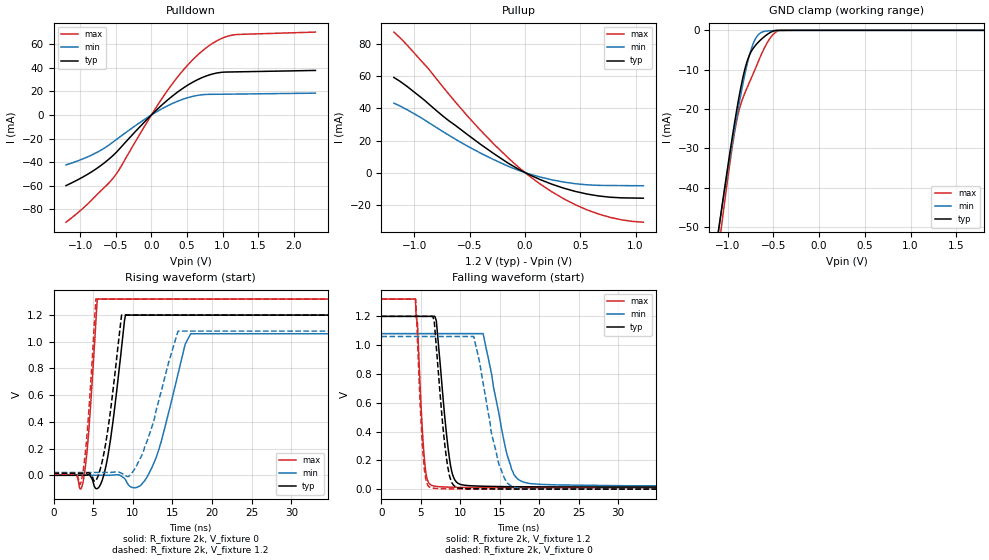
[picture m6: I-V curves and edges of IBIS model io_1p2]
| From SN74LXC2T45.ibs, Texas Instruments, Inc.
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[Model]   io_1p2
Model_type  I/O
Vinl=0.3
Vinh=0.9
Enable   Active-Low
Vref =   0
Rref =   2000
Cref =   15p
Vmeas =   0.6
| variable   typ   min   max
C_comp   6.34pF   5.61pF   7.15pF
| C_pullup   10.74pF   6.64pF   16.31pF
| C_pulldown   10.09pF   6.99pF   16.46pF
| C_tri-state   6.34pF   5.61pF   7.15pF
[Temperature Range]   25   125   -40
| Ambient temperature   25   85   -40
[Voltage range]   1.2   1.08   1.32
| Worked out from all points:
|   slope of the pulldown table from 0 to 0.18 V, typ, clamps not added: 17.6 ohm
|   slope of the pullup table from 0 to 0.18 V, typ, clamps not added: 32.4 ohm
|   GND clamp passes 1 mA (typ) near -0.56 V on its own axis
|   rising waveform, R_fixture 2k, V_fixture 0: 20-80 % time 1.47ns typ, 2.68ns min, 895ps max; typ from 0 V to 1.2 V
|   falling waveform, R_fixture 2k, V_fixture 1.2: 20-80 % time 1.23ns typ, 2.26ns min, 715ps max; typ from 1.2 V to 0.015 V
|   rising waveform, R_fixture 2k, V_fixture 1.2: 20-80 % time 1.51ns typ, 2.99ns min, 895ps max; typ from 0.015 V to 1.2 V
|   falling waveform, R_fixture 2k, V_fixture 0: 20-80 % time 1.19ns typ, 2.18ns min, 690ps max; typ from 1.2 V to 0 V
[GND Clamp]
| LXC8T245_IO_12
|   Voltage   I(typ)   I(min)   I(max)
-5.5V     -897.1mA   -831.9mA   -1.015A
-1.11V    -52.66mA   -52.33mA   -57.72mA
-1.08V    -47.7mA    -47.75mA   -52.14mA
-1.05V    -42.82mA   -43.24mA   -46.67mA
-915mV    -22.23mA   -23.93mA   -24.75mA
-835mV    -12.18mA   -13.81mA   -17.31mA
-785mV    -7.737mA   -8.436mA   -14.47mA
-735mV    -5.102mA   -4.277mA   -11.79mA
-645mV    -2.561mA   -727uA     -6.848mA
-530mV    -501.4uA   -105.7uA   -1.806mA
-430mV    -5.242uA   -35.39uA   -19.91uA
1.8V      23.18pA    30.38nA    510.2pA
[Pulldown]
| LXC8T245_IO_12
|   Voltage   I(typ)   I(min)   I(max)
-1.2V     -60.02mA   -42.43mA   -91.1mA
-835mV    -48.11mA   -33.91mA   -71.97mA
-655mV    -40.41mA   -27.94mA   -61.23mA
-525mV    -33.63mA   -22.34mA   -52.68mA
-430mV    -27.57mA   -18.06mA   -44.1mA
-110mV    -6.764mA   -4.321mA   -10.96mA
210mV     11.83mA    7.276mA    19.44mA
500mV     24.95mA    14.51mA    41.74mA
770mV     33.15mA    17.47mA    57.09mA
985mV     36.25mA    17.65mA    64.98mA
1.16V     36.61mA    17.76mA    68.13mA
2.305V    37.85mA    18.54mA    70.44mA
[Pullup]
| LXC8T245_IO_18
|   Voltage   I(typ)   I(min)   I(max)
-1.185V   59.29mA    43.25mA    87.57mA
-1.07V    53.91mA    39.34mA    79.78mA
-875mV    43.06mA    31.36mA    64.91mA
-625mV    29.2mA     20.66mA    43.65mA
-400mV    17.54mA    12.09mA    26.2mA
-150mV    5.788mA    3.92mA     9.044mA
35mV      -1.184mA   -766.3uA   -1.908mA
245mV     -7.266mA   -4.52mA    -12.05mA
350mV     -9.694mA   -5.885mA   -16.3mA
560mV     -13.33mA   -7.601mA   -23.19mA
770mV     -15.33mA   -8.028mA   -27.91mA
1.07V     -15.95mA   -8.192mA   -30.89mA
[Ramp]
| LXC8T245_IO_12
| variable   typ   min   max
dV/dt_r   0.72/2.3E-09   0.65/4.27E-09   0.79/1.1E-09
dV/dt_f   0.72/2.7E-09   0.65/4.1E-09   0.79/1.26E-9
R_load = 2k
[Rising Waveform]
| LXC8T245_IO_18
R_fixture =   2k
C_fixture =   0
L_fixture =   0
V_fixture =   0
V_fixture_min = 0
V_fixture_max = 0
|   Time   V(typ)   V(min)   V(max)
0s        267pV      9.22nV     2.33nV
3.7ns     -82.4uV    65.7nV     -57.2mV
4.47ns    4.06mV     356nV      352mV
5.52ns    -99.4mV    -2.34uV    1.32V
6.85ns    143mV      -106uV     1.32V
9.08ns    1.2V       -33.1mV    1.32V
10.7ns    1.2V       -85.3mV    1.32V
12.4ns    1.2V       58.1mV     1.32V
17.3ns    1.2V       1.06V      1.32V
50ns      1.2V       1.06V      1.32V
[Falling Waveform]
| LXC8T245_IO_18
R_fixture =   2k
C_fixture =   0
L_fixture =   0
V_fixture =   1.2
V_fixture_min = 1.08
V_fixture_max = 1.32
|   Time   V(typ)   V(min)   V(max)
0s        1.2V       1.08V      1.32V
4.31ns    1.2V       1.08V      1.32V
5.44ns    1.2V       1.08V      216mV
6.41ns    1.2V       1.08V      25.5mV
6.96ns    1.17V      1.08V      19.2mV
8.75ns    168mV      1.08V      13.8mV
9.92ns    35mV       1.08V      12.5mV
12.9ns    20.4mV     1.08V      11.2mV
17.7ns    16.8mV     56.8mV     10.4mV
50ns      14.9mV     21.8mV     9.87mV
[Rising Waveform]
| LXC8T245_IO_18
R_fixture =   2k
C_fixture =   0
L_fixture =   0
V_fixture =   1.2
V_fixture_min = 1.08
V_fixture_max = 1.32
|   Time   V(typ)   V(min)   V(max)
0s        14.8mV     21.5mV     9.86mV
3.47ns    14.7mV     21.5mV     -50.1mV
4.24ns    17.7mV     21.5mV     320mV
5.34ns    -39.9mV    21.5mV     1.32V
6.62ns    253mV      21.4mV     1.32V
8.58ns    1.2V       15.5mV     1.32V
9.59ns    1.2V       -3.12mV    1.32V
11.3ns    1.2V       171mV      1.32V
15.7ns    1.2V       1.08V      1.32V
50ns      1.2V       1.08V      1.32V
[Falling Waveform]
| LXC8T245_IO_18
R_fixture =   2k
C_fixture =   0
L_fixture =   0
V_fixture =   0
V_fixture_min = 0
V_fixture_max = 0
|   Time   V(typ)   V(min)   V(max)
0s        1.2V       1.06V      1.32V
4.32ns    1.2V       1.06V      1.32V
5.29ns    1.2V       1.06V      231mV
6.19ns    1.2V       1.06V      12mV
8.24ns    217mV      1.06V      2.51mV
9.37ns    16.8mV     1.06V      1.79mV
11.7ns    3.01mV     1.06V      1.11mV
14.9ns    1.48mV     171mV      682uV
16.7ns    1.13mV     16.2mV     530uV
50ns      52.8uV     208uV      5.46uV
